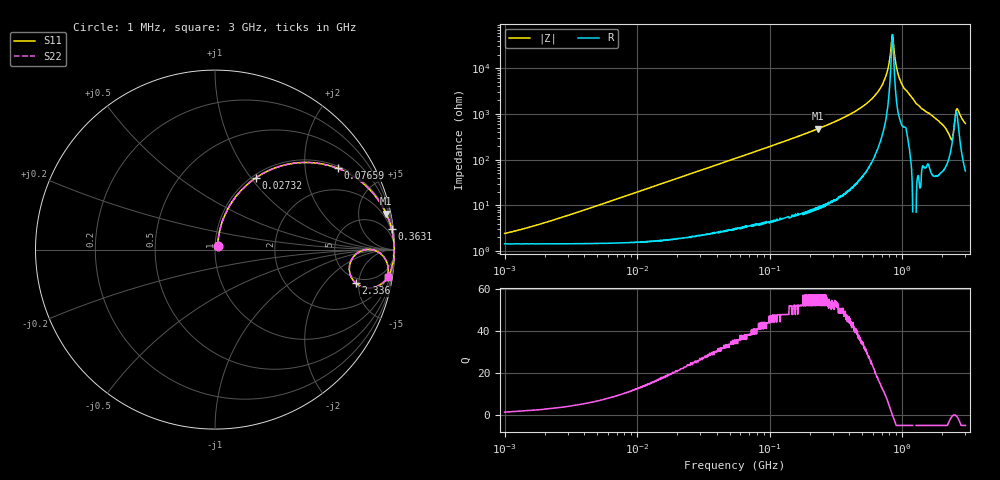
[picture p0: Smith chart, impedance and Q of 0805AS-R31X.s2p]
!s-Parameter Generated by FASTRON Sdn. Bhd.
!FASTRON P/N : 0805AS-R31X
!Keysight Technologies: E4991B_MY54100416_A.01.15
!Date: Mon Jun 15 12:53:55 2026
!Version  :Rev01  Mon Jun 15 12:53:55 2026
!Data & Calibration Information:
!Freq  S11  S21  S12  S22
!PortZ  Port1:50+j0  Port2:50+j0
!When reading reference impedance value at option line is always used.
! Remarks : This data is being provided solely for informational purposes.
# Hz S dB R 50
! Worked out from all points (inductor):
!   1601 points, 1 MHz to 3 GHz, reference 50 ohm
!   read as one part in series: L = 311 nH near 2.216 MHz
!   highest Q = 57.2 at 232.6 MHz (marker M1), where L = 327 nH
!   self-resonance near 841.6 MHz
!   S11 on the Smith chart (normalised r, x): 1 MHz: 1.03, +0.04; 27.32 MHz: 1.04, +1.06; 76.59 MHz: 1.07, +2.96; 363.1 MHz: 1, +17; 2.336 GHz: 4.30, -4.57; 3 GHz: 2, -12
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1000000  -32.40 52.6  -0.13 -1.1  -0.13 -1.1  -32.40 52.6
3804036  -22.60 74.7  -0.15 -4.2  -0.15 -4.2  -22.60 74.7
1.447069e7  -11.40 71.1  -0.47 -15.5  -0.47 -15.5  -11.40 71.1
2.732032e7  -6.72 60.3  -1.22 -27.5  -1.22 -27.5  -6.72 60.3
5.504702e7  -2.87 42.4  -3.41 -45.9  -3.41 -45.9  -2.87 42.4
7.658877e7  -1.73 33.6  -5.14 -55.0  -5.14 -55.0  -1.73 33.6
2.083556e8  -0.28 13.3  -12.80 -75.6  -12.80 -75.6  -0.28 13.3
2.326032e8  -0.22 11.8  -13.80 -77.2  -13.80 -77.2  -0.22 11.8
3.631036e8  -0.08 6.8  -18.60 -82.0  -18.60 -82.0  -0.08 6.8
6.296259e8  -0.02 2.2  -28.40 -84.9  -28.40 -84.9  -0.02 2.2
7.279565e8  -0.02 1.1  -34.30 -83.7  -34.30 -83.7  -0.02 1.1
7.925923e8  -0.01 0.5  -41.60 -78.1  -41.60 -78.1  -0.01 0.5
8.249649e8  -0.02 0.2  -49.20 -59.1  -49.20 -59.1  -0.02 0.2
8.501091e8  -0.02 -0.1  -54.00 25.8  -54.00 25.8  -0.02 -0.1
9.302341e8  -0.02 -0.7  -37.60 80.9  -37.60 80.9  -0.02 -0.7
1.02815e9  -0.03 -1.5  -31.50 80.6  -31.50 80.6  -0.03 -1.5
1.307284e9  -0.03 -3.6  -24.10 84.9  -24.10 84.9  -0.03 -3.6
1.970482e9  -0.22 -9.0  -16.10 76.2  -16.10 76.2  -0.22 -9.0
2.335937e9  -1.88 -13.4  -10.90 40.8  -10.90 40.8  -1.88 -13.4
2.480502e9  -1.30 0.1  -17.10 -0.3  -17.10 -0.3  -1.30 0.1
2.607784e9  -0.46 -3.1  -22.70 44.3  -22.70 44.3  -0.46 -3.1
3e9  -0.23 -9.0  -16.10 75.8  -16.10 75.8  -0.23 -9.0
